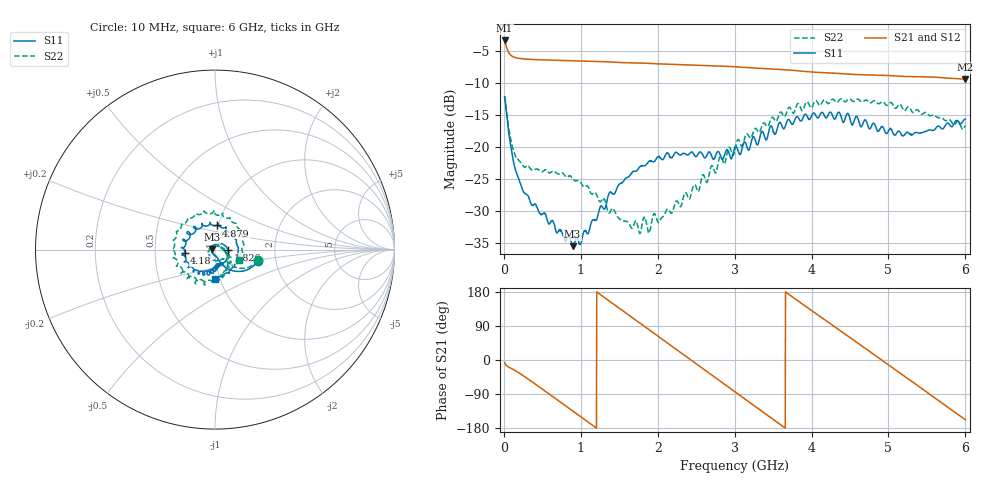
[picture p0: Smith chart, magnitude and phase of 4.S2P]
!Agilent Technologies,E5071C,MY46316741,A.11.02
!Date: Tue Oct 20 14:44:24 2020
!Data & Calibration Information:
!Freq	S11:SOLT4(ON)	S21:SOLT4(ON)	S12:SOLT4(ON)	S22:SOLT4(ON)
!PortZ  Port1:50+j0  Port2:50+j0
!Above PortZ is port z conversion or system Z0 setting when saving the data.
!When reading, reference impedance value at option line is always used.
# Hz S dB R 50
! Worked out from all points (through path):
!   1561 points, 10 MHz to 6 GHz, reference 50 ohm
!   highest |S21| = -3.34 dB at 10 MHz (marker M1); lowest = -9.4 dB at 6 GHz (marker M2)
!   group delay of S21, straight-line fit = 405 ps
!   lowest |S11| = -35.4 dB at 893.1 MHz (marker M3), VSWR 1.03, Z = 48.3 + j0.0834 ohm
!   |S11| at or under -10 dB: start of sweep to end of sweep
!   |S22| runs from -33.5 to -12.1 dB; largest |S21 - S12| = 0.0052
!   S11 on the Smith chart (normalised r, x): 10 MHz: 1.61, -0.23; 1.826 GHz: 1.15, -0.00; 4.18 GHz: 0.71, -0.03; 4.879 GHz: 0.98, +0.27; 6 GHz: 0.95, -0.32
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1e7  -12.12 -15.5  -3.34 -6.2  -3.41 -6.2  -12.08 -13.4
1.213526e8  -22.03 -66.4  -5.88 -24.9  -5.92 -24.8  -20.36 -44.6
2.480641e8  -26.78 -74.9  -6.21 -41.0  -6.24 -40.9  -22.86 -44.6
5.744423e8  -31.73 -108.1  -6.40 -87.5  -6.43 -87.5  -23.85 -66.8
8.93141e8  -35.43 177.1  -6.51 -134.1  -6.54 -134.2  -24.84 -101.9
1.012173e9  -34.52 137.1  -6.56 -151.6  -6.59 -151.7  -25.75 -116.8
1.36159e9  -27.43 57.8  -6.69 156.8  -6.72 156.8  -30.21 -173.5
1.764763e9  -23.08 4.3  -6.88 98.0  -6.89 97.8  -33.46 95.8
1.826199e9  -22.90 -0.7  -6.89 88.9  -6.92 88.8  -30.92 81.9
1.887635e9  -22.18 -9.1  -6.91 79.8  -6.94 79.6  -33.39 68.4
2.006667e9  -21.42 -20.9  -7.00 62.3  -7.02 62.3  -31.74 52.6
2.248571e9  -20.83 -44.3  -7.10 26.9  -7.12 26.7  -28.39 21.4
2.482795e9  -21.36 -60.9  -7.20 -7.3  -7.23 -7.6  -25.84 6.3
3.005e9  -19.99 -84.4  -7.45 -84.2  -7.49 -84.4  -20.37 -41.4
3.531045e9  -17.96 -110.8  -7.84 -161.2  -7.87 -161.4  -15.93 -85.6
4.007173e9  -14.91 -158.4  -8.27 129.7  -8.29 129.6  -13.75 -142.0
4.179962e9  -15.36 -173.9  -8.38 104.9  -8.42 104.8  -12.70 -156.9
4.490981e9  -15.17 150.0  -8.60 60.3  -8.63 60.0  -12.46 167.4
4.878795e9  -17.38 86.0  -8.76 4.7  -8.79 4.6  -13.20 122.9
5.001667e9  -17.44 65.4  -8.81 -13.2  -8.84 -13.3  -13.30 107.4
5.508513e9  -17.38 -20.9  -9.03 -86.2  -9.04 -86.3  -14.81 49.5
6e9  -15.61 -89.1  -9.40 -157.6  -9.40 -157.6  -16.58 -23.0
